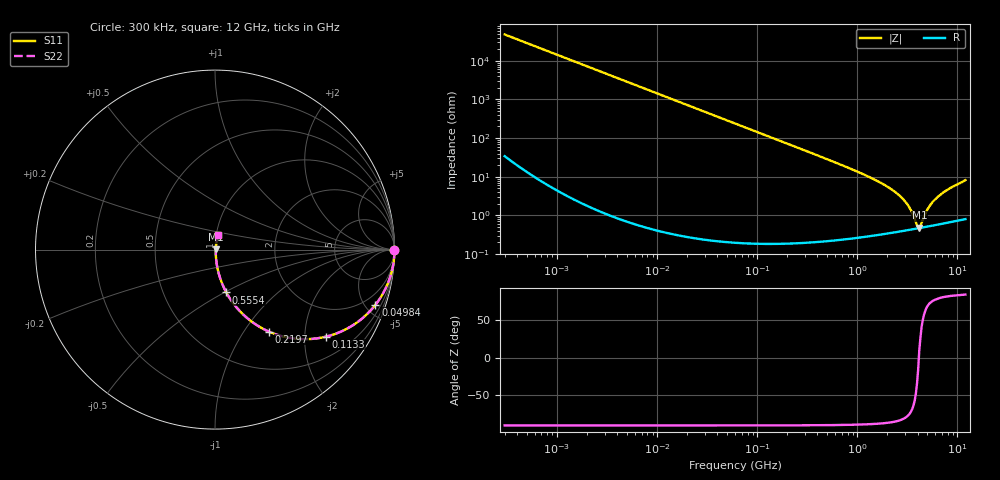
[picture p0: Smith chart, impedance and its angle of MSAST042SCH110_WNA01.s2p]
! MSAST042SCH110_WNA01  S-PARAMETER MODEL  ( General Type )
! Model Generated by TAIYO YUDEN Corporation (http://www.ty-top.com)
! Version 1.0
! TAIYO YUDEN Control No. 150820
! Copyright(c) 2015 TAIYO YUDEN CO.,LTD. All Rights Reserved.
! Product Description (link to TY-COMPAS)
! https://ds.yuden.co.jp/TYCOMPAS/or/detail?pn=MSAST042SCH110JWNA01&u=M
! Products Name : Multilayer Ceramic Capacitors
! Characteristics :
!  Capacitance : 11 pF , Rated Voltage : 25V , TCC : CH / C0H
!  Case Size : 0.4 x 0.2 / 0.016 x 0.008 [mm/inch] , Thickness : 0.2 / 0.008 [mm/inch]
!  (Conditions: Temperature = 25 degC , DC Bias Current/Voltage = 0A / 0V)
! External Node Assignments :
!  1  o---| |---o  2
! GND o---------o GND
! Frequency Range : 0.3MHz  -  12000MHz  [ 401 STEP ]
# MHz S RI R 50
! Freq[MHz].  S11 Real  S11 Imag  S21 Real  S21 Imag  S12 Real  S12 Imag  S22 Real  S22 Imag
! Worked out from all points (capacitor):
!   401 points, 300 kHz to 12 GHz, reference 50 ohm
!   read as one part in series: C = 11 pF near 316.3 kHz
!   lowest |Z| = 478 mohm at 4.159 GHz (marker M1)
!   series resonance near 4.114 GHz, so ESL is about 140 pH
!   S11 on the Smith chart (normalised r, x): 300 kHz: open; 49.84 MHz: 1.00, -5.79; 113.3 MHz: 1.00, -2.55; 219.7 MHz: 1.00, -1.31; 555.4 MHz: 1.00, -0.51; 12 GHz: 1.02, +0.16
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0.3  1 -0.00208  5.79e-06 0.00208  5.79e-06 0.00208  1 -0.00208
1.769972  0.9998 -0.0123  0.000153 0.0123  0.000153 0.0123  0.9998 -0.0123
10.44266  0.9948 -0.072  0.00523 0.072  0.00523 0.072  0.9948 -0.072
23.73947  0.9736 -0.1601  0.0264 0.1601  0.0264 0.1601  0.9736 -0.1601
49.84427  0.8933 -0.3084  0.1067 0.3084  0.1067 0.3084  0.8933 -0.3084
60  0.8524 -0.3543  0.1476 0.3543  0.1476 0.3543  0.8524 -0.3543
113.3117  0.6182 -0.4851  0.3818 0.4851  0.3818 0.4851  0.6182 -0.4851
219.7372  0.3008 -0.4572  0.6992 0.4572  0.6992 0.4572  0.3008 -0.4572
353.9943  0.142 -0.3466  0.858 0.3466  0.858 0.3466  0.142 -0.3466
555.3718  0.063 -0.2386  0.937 0.2386  0.937 0.2386  0.063 -0.2386
1229.528  0.014 -0.1052  0.986 0.1052  0.986 0.1052  0.014 -0.1052
2088.533  0.00605 -0.0509  0.9939 0.0509  0.9939 0.0509  0.00605 -0.0509
2581.562  0.00491 -0.0337  0.9951 0.0337  0.9951 0.0337  0.00491 -0.0337
3026.31  0.00452 -0.0218  0.9955 0.0218  0.9955 0.0218  0.00452 -0.0218
3454.93  0.00444 -0.0123  0.9956 0.0123  0.9956 0.0123  0.00444 -0.0123
3944.255  0.00457 -0.00308  0.9954 0.00308  0.9954 0.00308  0.00457 -0.00308
4158.869  0.00468 0.000887  0.9953 -0.000887  0.9953 -0.000887  0.00468 0.000887
4385.161  0.00481 0.00421  0.9952 -0.00421  0.9952 -0.00421  0.00481 0.00421
5140.631  0.00539 0.0148  0.9946 -0.0148  0.9946 -0.0148  0.00539 0.0148
6026.253  0.00624 0.0255  0.9938 -0.0255  0.9938 -0.0255  0.00624 0.0255
8064.993  0.00862 0.0462  0.9914 -0.0462  0.9914 -0.0462  0.00862 0.0462
12000  0.0144 0.0799  0.9856 -0.0799  0.9856 -0.0799  0.0144 0.0799
